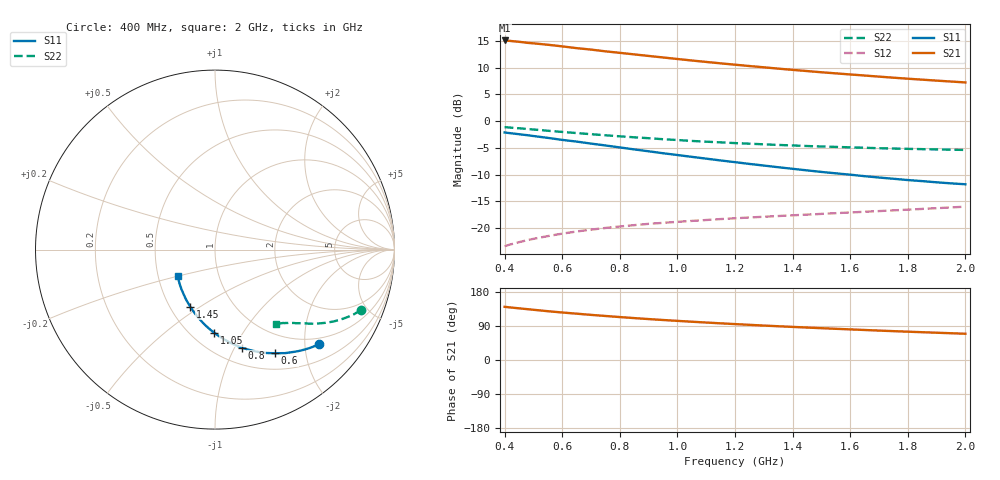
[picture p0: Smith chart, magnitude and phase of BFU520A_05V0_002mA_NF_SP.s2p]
! Filename:  P:\Prog\Test\Noise\ATS_data\Testdata_Net\06 Compressed Noise after Statistics\BFU520A_APG2013_30_A05_05p0V_002mA_NF_CM01_D.sf
! Date/Time: Wed 24/Apr/2013 20:06:17
! BFU520A_APG2013_30_A05_05p0V_1to20mA_NF_CM01_Bias2_R.sf
! Noise Parameter Data File
! BFU520A_APG2013_30_A05_05p0V_1to20mA_NF_CM01
! Date/time: Thu Apr 11 01:07:08 2013
! VAR V_out= 5.001000
! VAR I_out= 2.000000
! VAR V_in= 0.809700
! VAR I_in= 0.021505
! Device data file deembeded for feedlines and parallel
! Original file: \06 Compressed Noise after Statistics\BFU520A_APG2013_30_A05_05p0V_002mA_NF_CM01_R.sf
! Feed-files: PR017V01_150413_Feed1.s2p, PR017V01_150413_Feed2.s2p
! Parallel-file: PR017V01_150413_Par.s2p
# MHz S MA R 50
!  Freq-MHz  S11-mag  S11-arg  S21-mag  S21-arg  S12-mag  S12-arg  S22-mag  S22-arg
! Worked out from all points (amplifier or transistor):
!   37 points, 400 MHz to 2 GHz, reference 50 ohm
!   highest |S21| = 15.1 dB at 400 MHz (marker M1)
!   |S21| within 3 dB of that: start of sweep to 917.9 MHz
!   unconditionally stable (mu >= 1): nowhere
!   at 500 MHz: K = 0.35, MSG = 18.3 dB, |S12| = -22.0 dB
!   at 1.1 GHz: K = 0.70, MSG = 14.8 dB, |S12| = -18.5 dB
!   at 2 GHz: K = 0.99, MSG = 11.6 dB, |S12| = -16.0 dB
!   lowest NFmin = 0.54 dB at 440 MHz
!   S11 on the Smith chart (normalised r, x): 400 MHz: 0.85, -2.31; 600 MHz: 0.71, -1.49; 800 MHz: 0.67, -1.07; 1.05 GHz: 0.64, -0.76; 1.45 GHz: 0.63, -0.45; 2 GHz: 0.63, -0.20
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400  0.7829 -42.4  5.691 140.4  0.06758 66.0  0.8786 -22.5
420  0.7714 -44.4  5.634 138.6  0.07011 65.2  0.87 -23.4
440  0.7604 -46.2  5.564 137.1  0.0725 64.3  0.8616 -24.2
480  0.7383 -49.6  5.405 134.1  0.07698 62.7  0.8437 -25.8
500  0.7258 -51.5  5.351 132.5  0.07915 62.0  0.8354 -26.5
550  0.6973 -55.8  5.189 128.8  0.08397 60.3  0.813 -28.2
600  0.6678 -59.9  5.011 125.4  0.08853 58.9  0.7927 -29.7
650  0.6437 -63.5  4.822 122.3  0.09276 57.5  0.7736 -31.1
700  0.6165 -67.4  4.675 119.1  0.09649 56.5  0.7548 -32.4
750  0.5922 -70.9  4.502 116.2  0.1001 55.4  0.7376 -33.6
800  0.5675 -74.5  4.359 113.3  0.1033 54.6  0.7212 -34.6
850  0.5438 -77.9  4.214 110.6  0.1063 53.8  0.7059 -35.7
950  0.5009 -84.5  3.945 105.5  0.1117 52.7  0.6776 -37.5
1050  0.4633 -90.5  3.695 101.0  0.1165 52.0  0.6528 -39.1
1150  0.4286 -96.6  3.475 96.8  0.1212 51.5  0.6332 -40.5
1200  0.4132 -99.4  3.376 94.8  0.1232 51.5  0.6232 -41.1
1300  0.3842 -105.1  3.191 90.9  0.1274 51.4  0.607 -42.5
1450  0.3462 -113.6  2.943 85.6  0.1334 51.7  0.585 -44.3
1500  0.3348 -116.3  2.868 83.9  0.1355 51.9  0.5791 -44.8
1650  0.3054 -124.7  2.673 79.2  0.1419 52.7  0.5637 -46.6
1750  0.2889 -130.4  2.551 76.1  0.1462 53.3  0.5542 -47.7
2000  0.2565 -144.4  2.303 69.3  0.1584 55.0  0.5377 -50.6
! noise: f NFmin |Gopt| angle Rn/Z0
400  0.5636  0.5047  15.32  0.2132
460  0.5615  0.487  20.57  0.2075
600  0.6031  0.4814  27.1  0.2282
800  0.6107  0.4461  39.31  0.1773
1000  0.6531  0.4497  48.88  0.166
1200  0.7129  0.4299  57.8  0.1648
1400  0.7425  0.4013  70.25  0.1439
1600  0.7916  0.3508  81.67  0.1249
1800  0.7564  0.3053  96.14  0.1041
2000  0.7915  0.3036  104.4  0.1042
